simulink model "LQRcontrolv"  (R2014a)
settings: Solver=ode4  StartTime=0.0  StopTime=2  FixedStep=t0  RelTol=1e-3
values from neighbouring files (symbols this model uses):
  k1 = k(1)    [LQRposition.m]    (also in LQRvelocity.m)
  k2 = k(2)    [LQRposition.m]    (also in LQRvelocity.m)
  k3 = k(3)    [LQRvelocity.m]
  t0 = 0.0002    [LQRposition.m]    (also in LQRvelocity.m)
undefined symbols (not defined in the file or in its folder): ae, be, ce, de, DiscIntNeverNeededParam
libraries: slrtlib x4, xpcnilib x3, simulink x1, powerlib_meascontrol x1

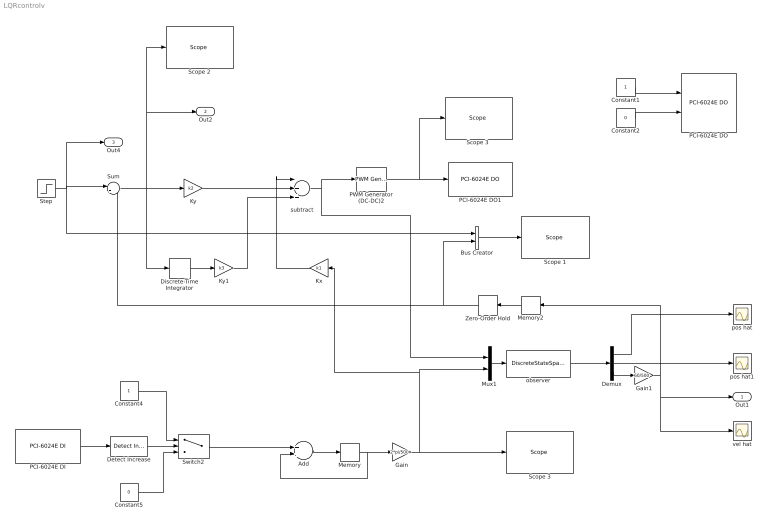
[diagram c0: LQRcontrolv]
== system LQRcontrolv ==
  Add : Sum
  Bus Creator : BusCreator  Inputs=2
  Constant1 : Constant
  Constant2 : Constant  Value=0
  Constant4 : Constant
  Constant5 : Constant  Value=0
  Demux : Demux  Outputs=3
  Detect Increase : simulink/Logic and Bit Operations/Detect Increase  vinit=0.0  InputProcessing=Inherited  OutDataTypeStr=boolean
  Discrete-Time Integrator : DiscreteIntegrator  SampleTime=t0  ICPrevOutput=DiscIntNeverNeededParam  ICPrevScaledInput=DiscIntNeverNeededParam
  Gain : Gain  Gain=2*pi/500
  Gain1 : Gain  Gain=60/500
  Kx : Gain  Gain=k1
  Ky : Gain  Gain=k2
  Ky1 : Gain  Gain=k3
  Memory : Memory  InheritSampleTime=on
  Memory2 : Memory
  Mux1 : Mux  Inputs=2
  PCI-6024E DI : xpcnilib/Digital Input/E Series/PCI-6024E DI  channel=[4]  sampletime=t0  slot=-1
  PCI-6024E DO : xpcnilib/Digital Output/E Series/PCI-6024E DO  channel=[1 2]  reset=[1]  initValue=[0]  sampletime=-1  slot=-1
  PCI-6024E DO1 : xpcnilib/Digital Output/E Series/PCI-6024E DO  channel=[3]  reset=[1]  initValue=[0]  sampletime=-1  slot=-1
  PWM Generator (DC-DC)2 : powerlib_meascontrol/Pulse & Signal Generators/PWM Generator (DC-DC)  Fsw=1000  Ts=t0
  Scope 1 : slrtlib/Displays and Logging/Scope   scopeno=1  scopetype=Target  autostart=on  viewmode=Graphical redraw  formatstr='%15.6f'  grid=on  ylimits=[0,0]  nosamples=2000  noprepostsamples=0  interleave=1  triggermode=FreeRun  triggersignal=1  trigsignalfromport=off  triggerlevel=0.0  triggerslope=Either  triggerscope=1  triggersample=0  filename=data.dat  mode=Lazy  writesize=512  autorestart=off  dynamicfilemode=off  maxwritefilesize=512*1024^2
  Scope 2 : slrtlib/Displays and Logging/Scope   scopeno=2  scopetype=Target  autostart=on  viewmode=Graphical redraw  formatstr='%15.6f'  grid=on  ylimits=[0,0]  nosamples=2000  noprepostsamples=0  interleave=1  triggermode=FreeRun  triggersignal=1  trigsignalfromport=off  triggerlevel=0.0  triggerslope=Either  triggerscope=1  triggersample=0  filename=data.dat  mode=Lazy  writesize=512  autorestart=off  dynamicfilemode=off  maxwritefilesize=512*1024^2
  Scope 3 : slrtlib/Displays and Logging/Scope   scopeno=4  scopetype=Target  autostart=on  viewmode=Graphical redraw  formatstr='%15.6f'  grid=on  ylimits=[0,0]  nosamples=2000  noprepostsamples=0  interleave=1  triggermode=FreeRun  triggersignal=1  trigsignalfromport=off  triggerlevel=0.0  triggerslope=Either  triggerscope=1  triggersample=0  filename=data.dat  mode=Lazy  writesize=512  autorestart=off  dynamicfilemode=off  maxwritefilesize=512*1024^2
  "Scope 3 " : slrtlib/Displays and Logging/Scope   scopeno=3  scopetype=Target  autostart=on  viewmode=Graphical redraw  formatstr='%15.6f'  grid=on  ylimits=[0,0]  nosamples=2000  noprepostsamples=0  interleave=1  triggermode=FreeRun  triggersignal=1  trigsignalfromport=off  triggerlevel=0.0  triggerslope=Either  triggerscope=1  triggersample=0  filename=data.dat  mode=Lazy  writesize=512  autorestart=off  dynamicfilemode=off  maxwritefilesize=512*1024^2
  Step : Step  Time=0.2  After=200  SampleTime=t0
  Sum : Sum  Inputs=|+-
  Switch2 : Switch  Criteria=u2 > Threshold
  Zero-Order Hold : ZeroOrderHold  SampleTime=t0
  observer : DiscreteStateSpace  A=ae  B=be  C=ce  D=de  X0=[0 0]  SampleTime=t0
  pos hat : Scope
  pos hat1 : Scope
  subtract : Sum  Inputs=-++
  vel hat : Scope
  Out1 : Outport
  Out2 : Outport  Port=2
  Out4 : Outport  Port=3
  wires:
  Memory/1 -> Gain/1, Add/2
  Constant1/1 -> PCI-6024E DO/1
  Constant2/1 -> PCI-6024E DO/2
  Add/1 -> Memory/1
  PCI-6024E DI/1 -> Detect Increase/1
  Sum/1 -> Discrete-Time Integrator/1, Ky/1, Scope 2/1, Out2/1
  Detect Increase/1 -> Switch2/2
  Constant4/1 -> Switch2/1
  Constant5/1 -> Switch2/3
  Step/1 -> Bus Creator/1, Out4/1, Sum/1
  Switch2/1 -> Add/1
  Mux1/1 -> observer/1
  observer/1 -> Demux/1
  Demux/1 -> pos hat/1
  Demux/2 -> pos hat1/1
  Bus Creator/1 -> Scope 1/1
  Discrete-Time Integrator/1 -> Ky1/1
  Ky1/1 -> subtract/3
  Ky/1 -> subtract/2
  Kx/1 -> subtract/1
  PWM Generator (DC-DC)2/1 -> PCI-6024E DO1/1, "Scope 3 "/1
  subtract/1 -> Mux1/1, PWM Generator (DC-DC)2/1
  Zero-Order Hold/1 -> Bus Creator/2, Sum/2
  Memory2/1 -> Zero-Order Hold/1
  Demux/3 -> Gain1/1
  Gain/1 -> Kx/1, Mux1/2, Scope 3/1
  Gain1/1 -> Out1/1, vel hat/1, Memory2/1
